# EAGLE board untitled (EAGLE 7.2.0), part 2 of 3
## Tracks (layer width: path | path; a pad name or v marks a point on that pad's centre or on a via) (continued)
N$28  (via drill 0.6) (continued)
  Top 0.406: R20.1 38.1,123.19 38.1,120.65 35.56,119.38 35.56,110.49 R18.1 | C7.2 66.04,110.49 63.5,107.95 v52.07,107.95 U1.18 52.07,101.6 54.61,99.06 U1.4 54.61,93.98 53.34,92.71 U$1.3 | R46.1 100.33,121.92 102.87,120.65 102.87,119.38 101.6,118.11 101.6,110.49 R44.1 | U2.4 109.22,99.06 109.22,104.46 U2.18 v107.95,109.22 | R67.1 146.05,123.19 146.05,110.49 R65.1 | v152.4,109.22 U3.18 152.4,102.87 154.94,100.33 U3.4 | R89.1 201.93,111.76 R87.1 208.28,109.22 v210.82,106.68 | v229.87,106.68 U4.18 229.87,102.87 232.41,100.33 U4.4
  Bottom 0.406: R18.1 38.1,107.95 v52.07,107.95 | U$1.3 56.83,88.9 R22.1 63.5,93.98 R24.2 | C7.2 93.98,111.76 96.52,109.22 R44.1 v107.95,109.22 109.22,110.49 146.05,110.49 R65.1 v152.4,109.22 153.67,110.49 203.2,110.49 R87.1 | v210.82,106.68 v229.87,106.68
N$29  (via drill 0.6)
  Top 0.406: v52.07,125.73 IC3.8 52.07,119.38 50.8,118.11 50.8,106.68 U1.19
  Bottom 0.406: R19.1 38.1,125.73 v52.07,125.73
N$30
  Top 0.406: R19.2 R20.2
  Bottom 0.406: R21.1 R20.2 41.91,124.46 IC3.13
N$31  (via drill 0.6)
  Top 0.406: IC2.6 v62.23,127 v57.15,127 57.15,124.46 R21.2
  Bottom 0.406: IC3.14 38.1,120.65 62.23,120.65 62.23,123.19 60.96,124.46 R21.2
N$32  (via drill 0.6)
  Top 0.406: IC3.2 39.37,113.03 43.18,109.22 43.18,102.87 44.45,101.6 v44.45,96.52
  Bottom 0.406: v44.45,96.52 48.26,96.52 U1.2
N$33
  Top 0.406: IC3.9 49.53,119.38 48.26,118.11 48.26,107.95 46.99,106.68 U1.20
N$34
  Top 0.406: C9.1 R25.2
  Bottom 0.61: IC3.4 45.72,115.57 57.15,115.57 C9.1
N$35
  Bottom 0.406: U$1.1 55.56,87.63 59.69,87.63 60.96,88.9 R22.2 R23.1
N$36
  Bottom 1.422: D12.C D10.A 123.19,149.86 IC4.15 118.11,149.86 118.11,162.56 121.92,167.64 X2.2
N$37
  Bottom 0.406: 138.43,149.86 IC5.1
  Bottom 1.422: IC5.1 133.35,149.86 D13.A D15.C | X2.3 124.46,162.56 127,160.02 137.16,160.02 138.43,158.75 138.43,149.86
N$38
  Top 0.406: C8.1 R26.2
  Bottom 0.406: C8.1 57.15,123.19 45.72,123.19 IC3.11
N$39
  Top 1.422: IC5.15 165.1,149.86 D14.A D16.C
  Bottom 1.422: X2.4 127,167.64 128.27,162.56 152.4,162.56 158.75,154.94 158.75,149.86 IC5.15
N$40
  Top 1.422: IC5.14 R30.1 166.37,154.94 D14.C
N$41
  Top 1.422: R29.1 IC5.2
  Bottom 1.422: D13.C 132.08,154.94 R29.1
N$42
  Top 1.422: D9.A 91.44,149.86 IC4.1
  Bottom 1.422: D11.C D9.A | IC4.1 97.79,151.13 97.79,157.48 99.06,158.75 110.49,158.75 119.38,168.91 X2.1
N$43
  Top 1.422: R28.1 IC4.14
  Bottom 1.422: D10.C 124.46,154.94 R28.1
N$44
  Top 1.422: D9.C 90.17,154.94 R27.1 IC4.2
N$45  (via drill 0.6)
  Top 0.406: IC4.13 R31.2 115.57,143.51 116.84,142.24 116.84,137.16 120.65,133.35 v123.19,133.35 | v153.67,133.35 153.67,137.16 154.94,138.43 IC5.13
  Bottom 0.406: v123.19,133.35 137.16,133.35 139.7,132.08 148.59,132.08 151.13,133.35 v153.67,133.35
N$46
  Top 0.406: R34.1 IC4.11
  Bottom 0.406: R34.1 110.49,142.24 110.49,139.7 R33.2
N$47  (via drill 0.6)
  Top 0.406: IC4.4 v102.87,152.4 | v106.68,152.4 107.95,151.13 107.95,142.24 109.22,140.97 R34.2 113.03,139.7 C11.2
  Bottom 0.406: v102.87,152.4 v106.68,152.4
N$48
  Top 0.406: C11.1 139.7,132.08 | C12.2 139.7,132.08 | 139.7,132.08 139.7,144.78 143.51,148.59 IC5.4
  Bottom 0.406: IC5.10 149.86,156.21 144.78,156.21 IC5.4
N$49
  Top 0.406: R35.2 IC5.11
N$50
  Top 0.406: OK1.1 R93.2
N$51
  Top 0.406: IC4.5 104.14,148.59 101.6,146.05 R36.2
N$52
  Bottom 0.406: R37.1 R36.1 C13.2
N$53
  Top 0.406: R38.2 IC4.7
  Bottom 0.406: R37.2 R38.2
N$54
  Bottom 0.406: C14.1 R38.1
N$55
  Top 0.406: C14.2 IC4.9
N$56
  Top 0.406: R39.2 142.24,146.05 144.78,148.59 IC5.5
N$57
  Top 0.406: C15.2 R39.1
  Bottom 0.406: R40.1 R39.1
N$58
  Top 0.406: IC5.7 R41.2
  Bottom 0.406: R40.2 R41.2
N$59
  Top 0.406: R41.1 C16.1
N$60
  Top 0.406: IC5.9 C16.2
N$61  (via drill 0.6)
  Top 0.406: IC4.6 v105.41,129.54 | R42.2 120.65,111.76 IC6.7 119.38,115.57 v119.38,127 118.11,128.27 115.57,128.27 v114.3,127 v111.76,129.54
  Bottom 0.406: v105.41,129.54 v111.76,129.54
N$62
  Top 0.406: R42.1 IC6.6 | R44.2 R43.2
  Bottom 0.406: R43.2 R42.1
N$63  (via drill 0.6)
  Top 0.406: R43.1 IC6.1 | U2.3 106.68,99.06 v106.68,111.76
  Bottom 0.406: v106.68,111.76 R43.1
N$64
  Bottom 0.406: R95.1 45.72,176.53 45.72,174.3 X1.9
N$65  (via drill 0.6)
  Top 0.406: IC6.8 116.84,123.19 v116.84,127 | U2.19 v105.41,110.49 | R45.1 99.06,125.73 v99.06,110.49
  Bottom 0.406: v116.84,127 116.84,128.27 101.6,128.27 R45.1 | v105.41,110.49 v99.06,110.49
N$66
  Top 0.406: R46.2 R45.2
  Bottom 0.406: IC6.13 105.41,123.19 106.68,124.46 R46.2 111.76,123.19 121.92,123.19 R47.1
N$67  (via drill 0.6)
  Top 0.406: IC5.6 146.05,132.08 143.51,129.54 129.54,129.54 v127,127 v121.92,127
  Bottom 0.406: 113.03,125.73 120.65,125.73 v121.92,127 | R47.2 113.03,125.73 | 113.03,125.73 109.22,125.73 107.95,127 105.41,127 102.87,124.46 IC6.14
N$68
  Top 0.406: IC6.2 104.14,113.03 104.14,99.06 U2.2
N$69  (via drill 0.6)
  Top 0.406: IC6.9 115.57,123.19 v109.22,123.19 | v100.33,120.65 100.33,109.22 102.87,106.68 U2.20
  Bottom 0.406: v109.22,123.19 109.22,120.65 v100.33,120.65
N$70
  Bottom 1.422: D20.C D18.A 207.01,149.86 200.66,149.86 | 200.66,149.86 IC7.15 | X3.2 210.82,166.37 205.74,161.29 204.47,161.29 200.66,157.48 200.66,149.86
N$71
  Bottom 0.406: R51.2 C19.1 124.46,116.84 113.03,116.84 IC6.4
N$72
  Bottom 0.406: R52.2 C18.1 123.19,120.65 111.76,120.65 IC6.11
N$73
  Bottom 1.422: D23.C D21.A 217.17,149.86 222.25,149.86 | IC8.1 222.25,149.86 | 222.25,149.86 222.25,158.75 219.71,161.29 215.9,161.29 213.36,165.1 X3.3
N$74
  Top 1.422: IC8.15 248.92,149.86 D22.A D24.C
  Bottom 1.422: IC8.15 242.57,149.86 242.57,157.48 240.03,160.02 227.33,160.02 223.52,163.83 217.17,163.83 215.9,166.37 X3.4
N$75
  Top 1.422: IC8.14 R50.1 250.19,154.94 D22.C
N$76
  Top 1.422: R49.1 IC8.2
  Bottom 1.422: R49.1 215.9,154.94 D21.C
N$77
  Top 1.422: D19.C D17.A 173.99,149.86 IC7.1
  Bottom 1.422: X3.1 204.47,163.83 201.93,163.83 196.85,158.75 182.88,158.75 180.34,156.21 180.34,149.86 IC7.1
N$78
  Top 1.422: IC7.14 R48.1
  Bottom 1.422: R48.1 208.28,154.94 D18.C
N$79
  Top 1.422: D17.C 173.99,154.94 R32.1 IC7.2
N$80  (via drill 0.6)
  Top 0.406: IC7.13 196.85,146.05 198.12,144.78 R53.2 204.47,143.51 207.01,140.97 v208.28,140.97 | v223.52,152.4 219.71,152.4 217.17,149.86 v217.17,142.24
  Bottom 0.406: IC8.13 236.22,152.4 v223.52,152.4 | v217.17,142.24 215.9,140.97 v208.28,140.97
N$81
  Top 0.406: IC7.11 R54.2 195.58,142.24 195.58,138.43 R55.1
N$82  (via drill 0.6)
  Top 0.406: C17.2 195.58,133.35 R55.2 193.04,135.89 193.04,139.7 190.5,142.24 190.5,151.13 v189.23,152.4
  Bottom 0.406: IC7.4 185.42,153.67 186.69,152.4 v189.23,152.4
N$83
  Top 0.406: IC8.4 224.79,152.4 224.79,134.62 | 224.79,134.62 C21.2 | 224.79,134.62 224.79,133.35 C17.1
  Bottom 0.406: IC8.10 233.68,156.21 228.6,156.21 IC8.4
N$84
  Top 0.406: IC8.11 R56.2
N$85
  Top 0.406: R57.2 184.15,146.05 185.42,147.32 186.69,147.32 IC7.5
N$86
  Bottom 0.406: R58.1 R57.1 C22.2
N$87
  Top 0.406: IC7.7 R59.2
  Bottom 0.406: R58.2 R59.2
N$88
  Top 0.406: C23.1 R59.1
N$89
  Top 0.406: C23.2 IC7.9
N$90
  Top 0.406: R60.2 226.06,144.78 228.6,148.59 IC8.5
N$91
  Top 0.406: R61.1 R60.1
  Bottom 0.406: C24.2 R60.1
N$92
  Top 0.406: R62.2 IC8.7
  Bottom 0.406: R62.2 R61.2
N$93
  Bottom 0.406: C25.1 R62.1
N$94
  Top 0.406: IC8.9 C25.2
N$95  (via drill 0.6)
  Top 0.406: IC7.6 187.96,138.43 182.88,133.35 175.26,133.35 172.72,130.81 161.29,130.81 160.02,129.54 v160.02,127 v165.1,127 163.83,125.73 163.83,115.57 IC9.7
  Bottom 0.406: R63.2 165.1,111.76 IC9.7
N$96
  Top 0.406: R65.2 R64.2
  Bottom 0.406: IC9.6 R63.1 R64.2
N$97
  Top 0.406: IC9.1 R64.1 148.59,110.49 148.59,101.6 U3.3
N$98  (via drill 0.6)
  Top 0.406: R66.1 158.75,125.73 162.56,125.73 IC9.8 | v151.13,123.51 151.13,120.65 149.86,120.65 148.59,119.38 148.59,113.03 149.86,111.76 U3.19
  Bottom 0.406: IC9.8 161.29,123.51 v151.13,123.51
N$99  (via drill 0.5 pad 0.41, 0.6)
  Top 0.406: v149.86,124.46 IC9.13
  Bottom 0.406: R68.1 R67.2 v149.86,124.46 R66.2
N$100  (via drill 0.6)
  Top 0.406: IC8.6 229.87,132.08 228.6,130.81 208.28,130.81 205.74,128.27 199.39,128.27 198.12,127 v171.45,127 | IC9.14 148.59,123.19 148.59,125.73 v151.13,125.73
  Bottom 0.406: R68.2 168.91,125.73 167.64,125.73 | 167.64,125.73 v167.64,127 v171.45,127 | v151.13,125.73 167.64,125.73
N$101
  Top 0.406: U3.2 151.13,96.52 153.03,96.52 153.67,97.47 153.67,99.06 151.13,101.6 151.13,113.03 IC9.2
N$102  (via drill 0.6)
  Top 0.406: U3.20 144.78,107.95 v144.78,123.19
  Bottom 0.406: IC9.9 160.02,122.87 152.4,122.87 151.45,122.56 150.81,122.56 150.18,122.87 149.86,123.19 v144.78,123.19
N$103
  Bottom 0.406: IC9.4 156.21,115.57 167.64,115.57 C27.1 R69.2
N$104
  Bottom 0.406: IC9.11 156.21,120.65 167.64,120.65 C26.1 R70.2
N$105
  Bottom 1.016: D26.A D28.C
  Bottom 1.422: D26.A 290.83,149.86 285.75,149.86 | 285.75,149.86 IC10.15 | 285.75,149.86 285.75,160.02 292.1,166.37 292.1,171.25 X4.2
N$106
  Bottom 1.016: D29.A D31.C
  Bottom 1.422: D29.A 300.99,149.86 306.07,149.86 | IC11.1 306.07,149.86 | 306.07,149.86 306.07,157.48 303.53,160.02 298.45,160.02 294.64,166.37 X4.3
N$107
  Top 1.016: D30.A D32.C
  Top 1.422: IC11.15 331.47,149.86 D30.A
  Bottom 1.422: IC11.15 326.39,149.86 326.39,157.48 325.12,158.75 309.88,158.75 306.07,162.56 299.72,162.56 297.18,166.37 X4.4
N$108
  Top 1.422: IC11.14 R74.1 332.74,154.94 D30.C
N$109
  Top 1.422: R73.1 IC11.2
  Bottom 1.422: R73.1 299.72,154.94 D29.C
N$110
  Top 1.422: IC10.1 265.43,151.13 257.81,151.13 D25.A
  Bottom 1.016: D27.C D25.A
  Bottom 1.422: IC10.1 265.43,149.86 265.43,156.21 267.97,158.75 279.4,158.75 X4.1
N$111
  Top 1.422: D26.C 292.1,154.94 R72.1 IC10.14
N$112
  Top 1.422: D25.C 257.81,154.94 R71.1 IC10.2
N$113  (via drill 0.6)
  Top 0.406: IC10.13 R75.2 283.21,143.51 v283.21,137.16 | IC11.13 v322.58,142.24
  Bottom 0.406: v322.58,142.24 308.61,142.24 307.34,140.97 307.34,138.43 304.8,135.89 288.29,135.89 287.02,137.16 v283.21,137.16
N$114
  Top 0.406: IC10.11 R76.2
  Bottom 0.406: R76.2 280.67,142.24 280.67,139.7 R77.1
N$115  (via drill 0.6)
  Top 0.406: IC10.4 270.51,148.59 267.97,144.78 v267.97,135.89 | C29.2 R77.2
  Bottom 0.406: v267.97,135.89 R77.2
N$116
  Top 0.406: C30.2 311.15,137.16 311.15,144.78 313.69,147.32 313.69,151.13 311.15,153.67 IC11.4
  Bottom 0.406: C29.1 306.07,132.08 C30.2 | IC11.10 317.5,153.67 312.42,153.67 IC11.4
N$117
  Top 0.406: IC11.11 R78.2
N$118
  Top 0.406: IC10.5 271.78,148.59 269.24,144.78 R79.2
N$119
  Bottom 0.406: R80.1 R79.1 C31.2
N$120
  Top 0.406: IC10.7 R81.2
  Bottom 0.406: R80.2 R81.2
N$121
  Bottom 0.406: R81.1 C32.1
N$122
  Top 0.406: IC10.9 C32.2
N$123
  Top 0.406: IC11.5 312.42,147.32 309.88,144.78 R82.2
N$124
  Bottom 0.406: R83.1 R82.1 C33.2
N$125
  Top 0.406: IC11.7 R84.2
  Bottom 0.406: R83.2 R84.2
N$126
  Bottom 0.406: C34.1 R84.1
N$127
  Top 0.406: IC11.9 C34.2
N$128  (via drill 0.6)
  Top 0.406: v219.71,111.76 IC12.7 220.98,115.57 220.98,125.73 v219.71,127 v214.63,127 | v273.05,128.27 IC10.6
  Bottom 0.406: v219.71,111.76 R85.2 | v214.63,127 214.63,128.27 215.9,129.54 271.78,129.54 v273.05,128.27
N$129
  Top 0.406: R86.2 R87.2 | IC12.6 R85.1
  Bottom 0.406: R86.2 R85.1
N$130  (via drill 0.6)
  Top 0.406: IC12.1 R86.1 208.28,111.76 v212.09,107.95 | v228.6,107.95 228.6,99.06 U4.3
  Bottom 0.406: v212.09,107.95 v228.6,107.95
N$131  (via drill 0.6)
  Top 0.406: IC12.8 218.44,120.65 v218.44,104.14
  Bottom 0.406: R88.1 203.2,125.73 203.2,120.65 218.44,120.65 IC12.8 | v218.44,104.14 226.06,104.14 U4.19
N$132
  Top 0.406: R88.2 R89.2 209.55,124.46 IC12.13
  Bottom 0.406: R89.2 R90.1
N$133  (via drill 0.6)
  Top 0.406: IC11.6 313.69,153.67 314.96,152.4 316.23,152.4 316.23,134.62 v306.07,125.73 | IC12.14 204.47,125.73 207.01,128.27 220.98,128.27 v222.25,127 223.52,127 | R90.2 224.79,125.73 223.52,127 | 223.52,127 v227.33,127
  Bottom 0.406: v227.33,127 274.32,127 276.86,125.73 v306.07,125.73
N$134  (via drill 0.6)
  Top 0.406: v227.33,102.87 U4.2
  Bottom 0.406: IC12.2 207.01,106.68 210.82,102.87 v227.33,102.87
N$135  (via drill 0.6)
  Top 0.406: IC12.9 215.9,120.65 v215.9,105.09
  Bottom 0.406: v215.9,105.09 U4.20
N$136
  Top 0.406: C36.1 R91.2
  Bottom 0.406: IC12.4 213.36,113.03 223.52,113.03 C36.1
N$137
  Top 0.406: C35.1 R92.2
  Bottom 0.406: IC12.11 213.36,123.19 223.52,123.19 C35.1
N$138
  Top 0.406: R94.1 24.13,172.72 24.13,176.53 40.64,176.53 40.64,174.09 X1.7
N$139  (via drill 0.6)
  Top 0.406: R97.1 106.05,177.17 115.57,177.17 v116.2,176.53
  Bottom 0.406: v116.2,176.53 127.3,176.53 X2.9
N$140  (via drill 0.6)
  Top 0.406: U2.14 118.11,102.87 119.38,101.6 v119.38,100.01 119.38,85.09 118.11,83.82 v118.11,77.47 | v62.23,100.01 U1.14 | v143.51,77.47 IC13.13 | RN1.2 IC16.2 | v106.68,77.47 v106.68,58.42
  Bottom 0.406: v119.38,100.01 v62.23,100.01 | v143.51,77.47 v118.11,77.47 v106.68,77.47 | IC23.52 v106.68,58.42 106.68,50.8 107.95,49.53 RN1.2
N$141
  Top 0.406: R98.1 233.68,176.53 232.41,177.8 215.8,177.8 X3.7
N$142
  Top 0.406: X3.9 220.98,173.99 222.25,172.72 222.25,168.91 223.52,167.64 233.68,167.64 234.95,168.91 R99.1
N$143  (via drill 0.6)
  Top 0.406: X4.7 293.27,175.36 292.1,176.53 278.13,176.53 275.59,173.99 R100.1 | JP2.1 267.97,177.8 270.51,175.26 v270.51,171.45
  Bottom 0.406: v270.51,171.45 271.78,170.18 274.32,170.18 R100.1
N$144
  Top 0.406: X4.9 298.45,174.3 298.45,175.26 295.91,177.8 276.86,177.8 R101.1
N$145  (via drill 0.6)
  Top 0.406: v243.84,148.59 243.84,144.78 240.03,140.97 v240.03,124.46
  Bottom 0.406: R99.2 243.84,162.56 v243.84,148.59 | v240.03,124.46 252.73,124.46 OK4.1
N$146  (via drill 0.6)
  Top 0.406: R98.2 246.38,176.53 250.19,172.72 250.19,166.37 251.46,165.1 v251.46,163.83 | v252.73,137.16 252.73,124.46 OK4.3
  Bottom 0.406: v251.46,163.83 252.73,161.29 v252.73,137.16
N$147  (via drill 0.6)
  Top 0.406: v11.43,147.32 11.43,144.78 15.24,140.97 v15.24,135.89
  Bottom 0.406: R95.2 21.59,175.26 21.59,162.56 20.32,161.29 13.97,161.29 12.7,160.02 12.7,153.67 11.43,152.4 v11.43,147.32 | v15.24,135.89 19.05,132.08 72.39,132.08 80.01,124.46 OK2.1
N$148
  Bottom 0.406: R94.2 15.24,171.45 13.97,170.18 7.62,170.18 5.08,167.64 5.08,135.89 10.16,130.81 71.12,130.81 74.93,127 OK2.3
N$149
  Bottom 0.406: R97.2 101.6,177.8 92.71,177.8 86.36,171.45 86.36,132.08 92.71,125.73 OK3.1
N$150  (via drill 0.6)
  Top 0.406: R96.2 88.9,171.45 v86.36,173.99
  Bottom 0.406: v86.36,173.99 85.09,172.72 85.09,130.81 86.36,129.54 86.36,127 87.63,125.73 OK3.3
N$151  (via drill 0.6)
  Top 0.406: R101.2 274.32,176.53 274.32,168.91 273.05,167.64 270.51,167.64 269.24,166.37 269.24,163.83 v265.43,163.83 | v264.16,148.59 265.43,147.32 265.43,125.73 OK5.1
  Bottom 0.406: v265.43,163.83 264.16,162.56 v264.16,148.59
N$152  (via drill 0.6)
  Top 0.406: R100.2 273.05,170.18 271.78,168.91 269.24,168.91 267.97,167.64 267.97,166.37 264.16,166.37 262.89,165.1 v262.89,163.83 | v262.89,148.59 262.89,147.32 264.16,146.05 OK5.3
  Bottom 0.406: v262.89,163.83 v262.89,148.59
N$153
  Bottom 1.676: F3.2A 16.51,124.46 11.43,119.38 7.62,119.38 5.08,116.84 B1.AC2
N$154
  Bottom 1.676: B1.AC1 10.16,109.22 12.7,106.68 12.7,99.06 X15.2
N$155  (via drill 0.6)
  Top 0.406: U2.13 120.65,102.87 121.92,101.6 v121.92,100.01 121.92,85.09 120.65,83.82 v120.65,78.74 | v64.77,100.97 U1.13 | IC13.14 v146.05,78.74 | RN1.3 IC16.3 | v105.41,78.74 v105.41,57.15 106.68,55.88 v106.68,46.99
  Bottom 0.406: v121.92,100.01 120.02,100.97 119.06,100.97 118.43,100.65 65.41,100.65 v64.77,100.97 | v146.05,78.74 v120.65,78.74 v105.41,78.74 | IC23.51 95.25,57.15 v105.41,57.15 | v106.68,46.99 RN1.3
N$156  (via drill 0.6)
  Top 0.406: U2.12 123.19,102.87 124.46,101.6 v124.46,100.01 124.46,85.09 123.19,83.82 v123.19,80.01 | v67.31,101.6 U1.12 | v148.59,80.01 IC13.15 | RN1.4 IC16.4 | v104.14,80.01 v104.14,55.88 105.41,54.61 105.41,45.72 v106.68,44.45
  Bottom 0.406: v124.46,100.01 121.92,101.6 118.75,101.6 118.11,101.28 67.95,101.28 v67.31,101.6 | v148.59,80.01 v123.19,80.01 v104.14,80.01 | IC23.50 v104.14,55.88 | v106.68,44.45 RN1.4
N$157  (via drill 0.6)
  Top 0.406: v127,95.57 v127,102.24 125.73,102.87 U2.11 | v151.13,95.57 IC13.17 | v69.85,102.24 U1.11 | IC16.5 RN1.5 107.31,41.91 104.78,44.45 104.78,52.71 v102.87,54.61 v102.87,95.57
  Bottom 0.406: v127,102.24 118.43,102.24 117.79,101.92 70.17,101.92 v69.85,102.24 | v151.13,95.57 146.68,95.57 146.05,96.2 130.49,96.2 129.86,95.57 v127,95.57 v102.87,95.57 | IC23.49 95.25,54.61 v102.87,54.61
N$158  (via drill 0.6)
  Top 0.406: U2.10 v125.73,94.62 | IC13.18 148.59,90.17 149.86,91.44 v149.86,94.62 | IC16.6 RN1.6 107.31,39.37 104.14,42.55 104.14,50.8 v102.23,53.34 101.6,53.98 v101.6,94.62
  Bottom 0.406: v149.86,94.62 149.54,94.93 130.81,94.93 130.49,94.62 v125.73,94.62 v101.6,94.62 84.14,94.62 81.28,97.79 U1.10 | IC23.48 v102.23,53.34
N$159  (via drill 0.6)
  Top 0.406: U2.9 v123.19,93.66 | v100.33,93.66 100.33,93.34 100.97,92.71 v100.97,52.07 103.5,49.53 103.5,40.64 107.31,36.83 RN1.7 IC16.7 | IC13.19 144.78,90.17 143.51,90.17 142.24,91.44 140.97,91.44 139.7,92.71 v139.7,93.66
  Bottom 0.406: U1.9 68.58,96.52 80.01,96.52 82.55,93.66 v100.33,93.66 v123.19,93.66 v139.7,93.66 | IC23.47 95.25,52.07 v100.97,52.07
N$160  (via drill 0.6)
  Top 0.406: U2.8 v120.65,91.44 | v62.23,95.25 U1.8 | IC16.8 RN1.8 107.31,34.29 102.87,38.74 102.87,47.63 v100.01,50.8 v100.01,91.44
  Bottom 0.406: IC13.20 140.97,91.44 v120.65,91.44 v100.01,91.44 81.92,91.44 78.42,95.25 v62.23,95.25 | IC23.46 v100.01,50.8
N$161  (via drill 0.6)
  Top 0.406: U2.7 v118.11,92.71 | IC13.21 v137.16,92.71 | RN1.9 IC16.9 | v99.06,92.71 v99.06,49.53 99.06,33.66 99.7,33.02 v100.33,33.02
  Bottom 0.406: v137.16,92.71 v118.11,92.71 v99.06,92.71 81.92,92.71 79.06,95.89 64.14,95.89 U1.7 | IC23.45 95.25,49.53 v99.06,49.53 | v100.33,33.02 101.6,31.75 RN1.9
N$162  (via drill 0.6)
  Top 0.406: IC17.18 186.69,101.6 v187.64,100.97 | U3.14 161.29,103.82 v161.29,102.87 161.29,90.17 160.66,88.58 160.66,61.6 v161.29,60.96 160.66,60.33 v160.66,39.37 | IC19.11 200.34,57.15 v200.34,58.42 | U4.14 240.03,102.87 238.76,101.6 238.76,91.44 237.49,90.17 v237.49,77.47 | IC21.3 226.06,76.2 224.47,74.61 v224.47,57.15 | v187.96,55.88 187.96,43.18 IC18.18
  Bottom 0.406: v187.64,100.97 186.69,101.6 162.56,101.6 v161.29,102.87 | v200.34,58.42 199.39,58.42 198.12,57.15 190.5,57.15 189.23,55.88 v187.96,55.88 IC14.13 | v237.49,77.47 233.68,77.47 232.41,76.2 IC21.3 | v224.47,57.15 223.52,57.15 220.98,54.61 209.55,54.61 208.28,55.88 IC19.11 | IC18.18 184.15,39.37 v160.66,39.37 | v161.29,60.96 156.21,60.96 154.94,62.23 IC20.2 RN4.2 114.3,62.23 107.95,68.58 IC23.60
N$163  (via drill 0.6)
  Top 0.406: IC18.17 v189.23,53.34 | v211.77,52.07 211.77,41.91 v209.55,39.37 | IC21.4 227.01,73.66 225.42,72.07 225.42,57.79 226.06,57.15 226.06,54.93 v225.74,54.61 | v239.39,74.93 240.03,75.57 240.03,90.17 241.3,91.44 241.3,101.6 242.57,102.87 U4.13 | v178.12,53.34 v178.12,58.42 | U3.13 165.1,101.6 163.83,100.33 163.83,93.03 164.46,92.39 164.46,64.14 163.51,63.18 163.51,58.74 v163.19,58.42
  Bottom 0.406: v189.23,53.34 IC14.14 v178.12,53.34 | IC19.12 208.28,53.34 209.55,52.07 v211.77,52.07 220.98,52.07 223.52,54.61 v225.74,54.61 | v209.55,39.37 204.47,39.37 203.2,40.64 190.5,40.64 IC18.17 | IC17.17 187.96,106.36 166.05,106.36 U3.13 | IC21.4 232.41,73.66 233.68,74.93 v239.39,74.93 | v178.12,58.42 v163.19,58.42 156.21,58.42 154.94,59.69 IC20.3 RN4.3 113.67,59.69 113.03,60.33 113.03,62.23 107.95,67.31 95.25,67.31 IC23.59
N$164  (via drill 0.6)
  Top 0.406: v190.5,50.8 v190.5,48.26 190.5,44.45 191.77,43.18 IC18.16 | IC21.7 226.38,63.82 226.38,58.1 227.01,57.47 227.01,53.34 v228.28,52.07 | U4.12 245.11,102.87 243.84,101.6 243.84,91.44 241.3,88.9 v241.3,67.31 | 174.62,104.14 v174.62,105.41 174.62,85.09 173.67,84.14 173.67,56.83 v172.72,55.88 v172.72,52.07
  Bottom 0.406: U3.12 168.91,104.14 175.26,104.14 | IC17.16 190.5,104.14 175.26,104.14 | v190.5,48.26 193.04,48.26 194.31,49.53 198.12,49.53 199.39,50.8 IC19.13 208.28,50.8 209.55,49.53 222.25,49.53 224.79,52.07 v228.28,52.07 | v190.5,50.8 IC14.15 173.99,50.8 v172.72,52.07 | v241.3,67.31 233.68,67.31 232.41,66.04 IC21.7 | 175.26,104.14 v174.62,105.41 | v172.72,55.88 156.21,55.88 154.94,57.15 IC20.4 RN4.4 124.46,57.15 123.83,57.79 113.67,57.79 112.39,59.06 112.39,61.6 107.95,66.04 IC23.58
N$165  (via drill 0.6, 0.6 pad 0.61)
  Top 0.406: IC17.15 194.31,102.87 193.04,101.6 193.04,92.71 194.31,91.44 v194.31,90.17 | v203.2,90.17 v203.2,49.53 | IC14.17 196.85,44.45 IC18.15 193.04,43.18 v193.04,52.07 | U3.11 v170.18,107.31 | IC21.8 227.33,62.23 227.33,58.1 227.96,57.47 227.96,55.88 229.87,53.98 v229.87,53.34 | U4.11 247.65,102.55 246.38,101.28 246.38,91.44 243.84,88.9 243.84,64.45 v243.52,64.14
  Bottom 0.406: v170.18,107.31 192.72,107.31 IC17.15 | v194.31,90.17 v203.2,90.17 | IC14.17 198.12,48.26 199.39,49.53 v203.2,49.53 208.28,49.53 209.55,48.26 IC19.15 222.88,48.26 225.11,50.48 228.92,50.48 229.87,51.44 v229.87,53.34 | v243.52,64.14 237.17,64.14 236.22,64.77 233.68,64.77 232.41,63.5 IC21.8 | v193.04,52.07 175.26,52.07 173.99,53.34 156.21,53.34 154.94,54.61 IC20.5 RN4.5 125.73,54.61 123.19,57.15 113.03,57.15 111.76,58.42 111.76,60.96 107.95,64.77 95.25,64.77 IC23.57
N$166  (via drill 0.6)
  Top 0.406: IC17.14 196.85,102.87 195.58,101.6 v195.58,91.44 | v204.47,91.44 v204.47,52.07 v204.47,45.72 | v232.41,54.93 235.27,54.93 237.49,57.15 237.49,62.23 IC21.13 | U4.10 247.65,90.17 245.11,87.63 v245.11,63.5 | U3.10 170.18,92.71 167.64,90.17 167.64,85.73 168.91,84.46 168.91,80.65 167.32,78.74 v167.32,50.8
  Bottom 0.406: v195.58,91.44 v204.47,91.44 | IC18.14 200.66,45.72 v204.47,45.72 | v232.41,54.93 229.23,54.93 227.01,53.34 223.84,53.34 221.3,50.8 IC19.16 209.55,50.8 208.28,52.07 v204.47,52.07 199.39,52.07 198.12,50.8 IC14.18 194.31,50.8 193.04,49.53 173.04,49.53 171.77,50.8 v167.32,50.8 156.21,50.8 154.94,52.07 IC20.6 RN4.6 125.73,52.07 124.46,53.34 124.46,54.61 122.56,56.52 112.39,56.52 111.12,57.79 111.12,60.33 107.95,63.5 IC23.56 | v245.11,63.5 244.47,62.87 236.85,62.87 IC21.13
N$167  (via drill 0.6)
  Top 0.406: IC17.13 199.39,102.87 200.66,101.6 203.2,101.6 205.74,99.06 v205.74,54.61 v205.74,44.45 | IC21.14 234.95,64.77 234.95,57.47 234.31,56.83 v231.77,56.83 | U4.9 245.11,91.44 242.57,88.9 242.57,66.68 v242.25,66.04 | v191.77,46.99 v191.77,53.02 | U3.9 167.64,94.62 166.37,93.34 166.37,63.5 164.78,61.91 164.78,49.85 165.1,49.53 v165.1,48.26
  Bottom 0.406: IC18.13 201.93,44.45 v205.74,44.45 | v231.77,56.83 228.92,56.83 227.01,55.56 223.2,55.56 220.98,53.34 IC19.17 209.55,53.34 208.28,54.61 v205.74,54.61 199.39,54.61 198.12,53.34 IC14.19 193.99,53.34 192.72,53.02 v191.77,53.02 | v242.25,66.04 240.66,66.04 240.03,66.68 237.17,66.68 IC21.14 | v191.77,46.99 179.07,46.99 177.8,48.26 v165.1,48.26 156.21,48.26 154.94,49.53 IC20.7 RN4.7 130.17,49.53 128.91,50.8 125.73,50.8 123.83,52.71 123.83,53.98 121.92,55.88 111.76,55.88 110.49,57.15 110.49,59.69 107.95,62.23 95.25,62.23 IC23.55
N$168  (via drill 0.6)
  Top 0.406: IC17.12 201.93,104.14 203.2,102.87 204.47,102.87 207.01,100.33 v207.01,57.15 v207.01,41.91 | v223.2,58.1 v223.2,72.39 | U4.8 242.57,91.44 240.66,89.54 240.66,73.98 v240.35,73.66 | v195.58,45.72 195.58,54.61 IC14.20 | v164.15,45.72 164.15,62.55 165.42,63.82 165.42,97.47 U3.8
  Bottom 0.406: IC14.20 198.12,55.88 199.39,57.15 v207.01,57.15 208.28,57.15 209.55,55.88 IC19.18 220.66,55.88 222.88,58.1 v223.2,58.1 | IC18.12 203.2,43.18 205.74,43.18 v207.01,41.91 | v223.2,72.39 232.41,72.39 233.68,73.66 IC21.17 v240.35,73.66 | v195.58,45.72 v164.15,45.72 156.21,45.72 154.94,46.99 IC20.8 RN4.8 128.27,46.99 123.19,52.07 123.19,53.34 121.28,55.25 111.12,55.25 109.86,56.52 109.86,59.06 107.95,60.96 IC23.54
N$169  (via drill 0.6)
  Top 0.406: v209.55,59.69 v209.55,41.91 | U4.7 240.03,91.44 238.76,90.17 238.76,76.84 v238.12,76.2 | v221.93,74.93 v221.93,60.96 | v163.83,102.87 162.56,101.6 U3.7 | v152.4,94.3 152.4,80.01 149.86,77.47 149.86,71.12 148.59,69.85 148.59,46.99 RN4.9 | v194.31,43.5 194.31,55.88 IC14.21 | v107.95,59.06 v107.95,43.18
  Bottom 0.406: IC17.11 204.47,102.87 v163.83,102.87 | v209.55,41.91 208.6,40.64 205.42,40.64 IC18.11 | IC14.21 198.12,58.42 199.39,59.69 v209.55,59.69 210.82,58.42 IC19.19 219.39,58.42 v221.93,60.96 | v238.12,76.2 IC21.18 233.68,76.2 232.41,74.93 v221.93,74.93 | U3.7 162.56,96.52 160.34,94.3 v152.4,94.3 | v194.31,43.5 193.67,43.18 156.21,43.18 154.94,44.45 IC20.9 RN4.9 133.35,44.45 132.08,43.18 v107.95,43.18 | IC23.53 95.25,59.69 107.31,59.69 v107.95,59.06
N$170  (via drill 0.6)
  Top 0.406: IC21.11 236.22,57.15 234.95,55.88 231.77,55.88 230.82,54.93 230.82,52.39 228.92,50.48 224.47,50.48 219.71,45.72 v219.71,26.67
  Bottom 0.406: v219.71,26.67 219.71,24.13 217.8,22.23 170.81,22.23 168.59,20 162.56,20 162.56,17.78 160.02,17.78 IC15.5
N$171  (via drill 0.6)
  Top 0.406: U4.6 237.49,91.44 236.22,90.17 v236.22,89.85 | v219.71,88.9 219.71,83.82 220.98,82.55 220.98,80.01 220.34,78.74 v220.34,62.23 | U3.6 v160.02,91.44 | v140.97,60.96 IC13.12 140.97,82.55 142.24,83.82 142.24,90.17 140.97,90.17 v138.43,92.71 v138.43,97.79
  Bottom 0.406: v236.22,89.85 220.66,89.85 v219.71,88.9 | v220.34,62.23 212.09,62.23 210.82,60.96 IC19.9 199.39,60.96 198.12,59.69 187.96,59.69 186.69,58.42 IC14.12 179.7,58.42 178.75,59.37 162.88,59.37 162.56,59.69 IC20.18 156.21,59.69 154.94,60.96 v140.97,60.96 | v138.43,97.79 115.57,97.79 | U1.6 60.96,99.06 63.5,99.06 63.82,99.38 113.98,99.38 115.57,97.79 | 115.57,97.79 U2.6 | v138.43,92.71 138.75,92.39 141.29,92.39 143.51,90.17 158.75,90.17 v160.02,91.44
N$172
  Top 0.406: U3.15 160.02,101.6 158.75,100.33 158.75,85.09 160.02,83.82 160.02,41.59 159.7,41.28 159.7,39.37 158.75,38.42 158.75,34.29 157.48,34.29 157.48,22.86 IC15.10
  Bottom 0.406: U1.15 60.64,106.36 159.07,106.36 U3.15
N$173  (via drill 0.6)
  Top 0.406: U2.15 115.57,102.87 116.84,101.6 116.84,86.36 115.57,85.09 115.57,76.2 114.3,74.93 v114.3,60.96 | U4.15 233.68,101.28 233.68,95.25 v229.87,91.44 | v212.09,91.44 212.09,53.34 213.36,52.07 213.36,42.23 v209.55,37.78 | IC15.9 v156.21,31.75 | v137.48,31.75 v137.48,60.96
  Bottom 0.406: v229.87,91.44 v212.09,91.44 | v209.55,37.78 209.55,35.56 207.01,33.02 187.01,33.02 185.74,32.39 174.94,32.39 173.99,33.02 165.1,33.02 163.83,31.75 v156.21,31.75 v137.48,31.75 | v137.48,60.96 v114.3,60.96
N$174  (via drill 0.6)
  Top 0.406: U2.16 113.03,102.87 114.3,101.6 114.3,92.71 115.57,91.44 IC13.31 115.57,87.63 114.3,86.36 114.3,77.15 v113.35,76.2 | IC23.41 91.44,46.67 90.17,47.94 v90.17,76.2
  Bottom 0.406: U1.16 58.42,104.14 69.85,104.14 71.12,102.55 112.39,102.55 113.03,103.19 U2.16 | v113.35,76.2 v90.17,76.2
N$175  (via drill 0.6)
  Top 0.406: U4.16 234.95,106.68 238.76,106.68 238.76,104.14 236.22,101.6 236.22,92.71 234.95,91.44 v234.95,88.9 | v228.6,88.9 228.6,86.36 226.06,83.82 v226.06,78.74 | v218.44,78.74 v218.44,86.36 | U3.16 157.48,104.14 156.21,102.87 v156.21,88.9 v156.21,85.09 | v97.79,90.17 98.42,89.54 98.42,72.39 95.25,69.22 95.25,68.26 94.3,67.31 93.34,67.31 92.08,66.04 v92.08,50.8 | v128.27,10.16 128.27,13.97 127.95,14.29 127.95,21.27 127.64,21.59 v127.64,27.31 | v99.7,27.62 99.7,28.26 97.16,30.8 97.16,39.69 92.39,44.45 90.17,44.45 90.17,46.99 IC23.40 v88.9,50.8
  Bottom 0.406: v234.95,88.9 v228.6,88.9 | v226.06,78.74 v218.44,78.74 IC19.27 | v218.44,86.36 217.17,83.82 IC14.31 184.15,83.82 182.88,85.09 171.45,85.09 168.91,82.55 158.75,82.55 v156.21,85.09 | v156.21,88.9 153.67,88.9 152.4,87.63 137.16,87.63 137.16,90.17 v97.79,90.17 | IC15.28 142.24,8.89 141.29,9.84 133.35,9.84 133.03,9.53 131.76,9.53 131.13,10.16 v128.27,10.16 | v127.64,27.31 100.01,27.31 v99.7,27.62 | v92.08,50.8 v88.9,50.8
N$176  (via drill 0.6)
  Top 0.406: IC13.4 120.65,54.61 119.38,53.34 119.38,38.1 IC16.14 | v136.52,36.83 v136.52,23.5
  Bottom 0.406: IC14.4 177.8,78.74 173.67,74.61 163.51,74.61 163.19,74.93 121.92,74.93 IC13.4 | IC16.14 v136.52,36.83 | v136.52,23.5 136.52,23.18 140.65,19.05 IC15.20
N$177  (via drill 0.6)
  Top 0.406: IC13.5 v123.19,69.85 v123.19,49.53 123.19,40.64 125.41,38.42 v125.41,24.45 | v132.4,24.45 v132.4,10.48
  Bottom 0.406: IC19.25 212.09,73.66 208.28,77.47 187.96,77.47 186.69,76.2 IC14.5 177.8,76.2 174.62,73.03 171.77,73.03 170.5,71.76 169.23,71.76 167.64,70.17 123.51,70.17 v123.19,69.85 | v125.41,24.45 v132.4,24.45 | IC15.27 144.78,10.16 142.24,10.16 141.6,10.8 133.03,10.8 v132.4,10.48 | IC16.19 v123.19,49.53
N$178  (via drill 0.6)
  Top 0.406: v171.45,83.82 170.18,82.55 v170.18,76.2
  Bottom 0.406: IC14.2 R102.1 v171.45,83.82 | v170.18,76.2 116.84,76.2 115.57,74.93 IC13.2 115.57,72.39 114.3,71.12 95.89,71.12 94.61,69.85 93.66,69.85 92.71,68.9 92.71,67.95 90.49,65.72 83.5,65.72 81.28,63.5 IC23.34
N$179  (via drill 0.6)
  Top 0.406: v171.45,81.28 v171.45,76.2
  Bottom 0.406: IC14.3 R103.1 v171.45,81.28 | v171.45,76.2 171.45,75.88 170.81,75.25 163.83,75.25 163.51,75.57 118.75,75.57 118.11,74.93 IC13.3 116.52,72.07 116.52,67.63 SV3.2
N$180  (via drill 0.6)
  Top 0.406: IC13.29 120.65,85.09 119.38,83.82 v119.38,71.12 119.38,54.61 118.11,53.34 118.11,34.29 IC16.12 | v133.67,31.75 v133.67,24.45
  Bottom 0.406: IC14.29 187.96,78.74 186.69,77.47 177.8,77.47 173.99,73.66 171.45,73.66 170.18,72.39 168.91,72.39 167.64,71.12 v119.38,71.12 | IC16.12 v133.67,31.75 | v133.67,24.45 140.97,24.45 IC15.18
N$181  (via drill 0.6)
  Top 0.406: IC13.28 123.19,85.09 121.92,83.82 v121.92,68.9 121.92,35.56 IC16.13 | v143.51,24.13 138.43,29.21 v138.43,34.29
  Bottom 0.406: IC14.28 187.96,76.2 186.69,74.93 177.8,74.93 175.26,72.39 172.08,72.39 170.81,71.12 169.54,71.12 167.96,69.53 124.14,69.53 123.19,68.9 v121.92,68.9 | IC15.19 v143.51,24.13 | v138.43,34.29 IC16.13
N$182  (via drill 0.6)
  Top 0.406: 125.73,63.5 IC13.6 v125.73,45.72 | IC14.6 182.88,72.39 182.88,49.53 180.34,49.53 v180.34,44.45
  Bottom 0.406: IC14.6 186.69,73.66 187.96,74.93 199.39,74.93 200.66,76.2 IC19.3 | v180.34,44.45 IC20.12 156.21,44.45 154.94,45.72 v125.73,45.72
N$183  (via drill 0.6)
  Top 0.406: IC13.25 130.81,85.09 129.54,83.82 v129.54,66.68 v129.54,39.37 v129.54,23.5
  Bottom 0.406: IC14.25 187.96,68.58 186.69,67.31 130.17,67.31 v129.54,66.68 | v129.54,23.5 130.81,23.5 131.44,23.18 135.57,23.18 140.97,17.78 144.78,17.78 IC15.21 | IC16.15 v129.54,39.37
N$184  (via drill 0.6)
  Top 0.406: IC13.23 135.89,85.09 134.62,83.82 v134.62,41.91 v134.62,22.23 | v162.56,64.77 v162.56,87
  Bottom 0.406: IC14.23 187.96,63.5 186.69,62.23 165.1,62.23 v162.56,64.77 | v162.56,87 154.3,87 153.67,86.36 135.89,86.36 IC13.23 | v134.62,22.23 135.57,22.23 141.29,16.51 IC15.22 | IC16.16 v134.62,41.91
N$185  (via drill 0.6)
  Top 0.406: v208.28,72.39 v208.28,63.5 | IC13.26 128.27,85.09 127,83.82 v127,67.31 127,46.04 v128.59,44.45 128.59,21.91 128.91,21.59 v128.91,15.24
  Bottom 0.406: IC19.21 v208.28,63.5 | v208.28,72.39 200.66,72.39 199.39,71.12 IC14.26 187.96,71.12 186.69,69.85 170.18,69.85 168.59,68.26 127.95,68.26 v127,67.31 | IC15.25 144.78,15.24 v128.91,15.24 | IC16.17 v128.59,44.45
N$186  (via drill 0.6)
  Top 0.406: IC13.27 125.73,85.09 124.46,83.82 v124.46,68.26 v124.46,46.99 124.46,44.45 126.36,42.55 126.36,20.64 126.68,20.32 126.68,13.97 127,13.65 v127,10.8
  Bottom 0.406: IC19.24 212.09,71.12 208.28,74.93 200.66,74.93 199.39,73.66 IC14.27 187.96,73.66 186.69,72.39 176.53,72.39 175.89,71.76 172.4,71.76 171.13,70.49 169.86,70.49 168.27,68.9 125.1,68.9 v124.46,68.26 | IC15.26 143.19,11.75 127.95,11.75 v127,10.8 | IC16.18 v124.46,46.99
N$187  (via drill 0.6)
  Top 0.406: 128.27,63.5 IC13.7 v128.27,48.9 | 177.8,69.85 v177.8,71.12 177.8,60.96 177.16,60.33 v177.16,46.99
  Bottom 0.406: IC19.4 200.66,73.66 199.39,72.39 187.96,72.39 186.69,71.12 IC14.7 v177.8,71.12 | v177.16,46.99 IC20.13 156.21,46.99 154.94,48.26 128.91,48.26 v128.27,48.9
N$188  (via drill 0.6)
  Top 0.406: IC13.8 v130.81,50.8 | v171.45,68.58 v171.45,49.53
  Bottom 0.406: IC19.5 200.66,71.12 199.39,69.85 187.96,69.85 186.69,68.58 IC14.8 v171.45,68.58 | v171.45,49.53 IC20.14 156.21,49.53 154.94,50.8 v130.81,50.8
N$189  (via drill 0.6)
  Top 0.406: IC13.9 v133.35,53.34 | v170.18,66.04 v170.18,52.07
  Bottom 0.406: IC19.6 200.66,68.58 199.39,67.31 187.96,67.31 186.69,66.04 IC14.9 v170.18,66.04 | v170.18,52.07 IC20.15 156.21,52.07 154.94,53.34 v133.35,53.34
N$190  (via drill 0.6)
  Top 0.406: IC13.10 v135.89,55.88 | v168.91,63.5 v168.91,54.61
  Bottom 0.406: IC19.7 200.66,66.04 199.39,64.77 187.96,64.77 186.69,63.5 IC14.10 v168.91,63.5 | v168.91,54.61 IC20.16 156.21,54.61 154.94,55.88 v135.89,55.88
N$191  (via drill 0.6)
  Top 0.406: IC13.11 v138.43,58.42 | v166.05,60.96 v166.05,57.15
  Bottom 0.406: IC19.8 200.66,63.5 199.39,62.23 187.96,62.23 186.69,60.96 IC14.11 v166.05,60.96 | v166.05,57.15 IC20.17 156.21,57.15 154.94,58.42 v138.43,58.42
N$192  (via drill 0.6)
  Top 0.406: IC13.24 133.35,85.09 132.08,83.82 v132.08,66.04 | v142.24,66.04 v142.24,41.91 | IC18.19 186.69,44.45 186.69,66.04 187.96,67.31 | IC17.19 184.15,100.33 185.42,99.06 185.42,91.44 187.96,88.9 187.96,67.31 | IC14.24 195.58,67.31 187.96,67.31
  Bottom 0.406: IC14.24 199.39,66.04 200.66,67.31 209.55,67.31 210.82,66.04 IC19.22 | v132.08,66.04 v142.24,66.04 | v142.24,41.91 148.59,41.91 149.86,40.64 182.88,40.64 IC18.19
N$193  (via drill 0.6)
  other vias: 93.98,165.1
N$194
  pour Top: 173.99,163.19 175.89,163.19 175.89,164.78 173.99,164.78
N$195  (via drill 0.6)
  other vias: 190.5,163.83
N$196
  Bottom 1.676: X15.6 11.43,80.01 39.37,80.01 40.64,81.28 44.45,81.28 B2.AC1
N$197  (via drill 0.6)
  Top 0.406: IC17.9 RN2.9 | OK5.8 267.97,113.03 265.43,113.03 264.16,111.76 261.62,111.76 260.35,107.95 260.35,97.79 v256.54,93.98
  Bottom 0.406: v256.54,93.98 RN2.9
N$198  (via drill 0.6)
  Top 0.406: IC17.8 RN2.8 | OK5.6 262.89,113.03 260.35,113.03 257.81,109.22 257.81,97.79 v252.73,92.71
  Bottom 0.406: v252.73,92.71 200.66,92.71 RN2.8
N$199  (via drill 0.6)
  Top 0.406: IC17.7 RN2.7 | OK4.8 254,113.03 254,97.79 v252.09,95.89
  Bottom 0.406: v252.09,95.89 198.44,95.89 RN2.7
N$200  (via drill 0.6)
  Top 0.406: IC17.6 RN2.6 | OK4.6 250.19,111.76 251.46,110.49 v251.46,97.79
  Bottom 0.406: v251.46,97.79 250.19,96.52 195.58,96.52 IC17.6
N$201  (via drill 0.6)
  Top 0.406: RN2.5 IC17.5 191.77,101.6 190.5,102.87 v190.5,112.4 | OK3.8 v92.71,109.22 | v143.51,109.22 v143.51,115.57
  Bottom 0.254: v92.71,109.22 93.34,108.27 143.51,108.27 v143.51,109.22 | v143.51,115.57 143.51,116.21 172.72,116.21 172.72,113.67 173.99,112.4 v190.5,112.4
N$202  (via drill 0.6)
  Top 0.406: OK3.6 v87.63,109.22 | v187.96,109.54 187.96,102.87 189.23,101.6 IC17.4 RN2.4 v189.23,90.17 | v181.61,90.17 179.07,87.63 179.07,52.07 178.43,51.44 178.43,46.36 177.8,45.72 v177.8,41.91 | v167.64,41.91 167,41.28 167,29.85 166.37,29.21 v166.37,8.89
  Bottom 0.254: v87.63,109.22 88.9,107.95 168.27,107.95 169.86,109.54 v187.96,109.54
  Bottom 0.406: v189.23,90.17 v181.61,90.17 | v177.8,41.91 v167.64,41.91 | v166.37,8.89 165.1,8.89 162.56,6.35 IC15.39
N$203  (via drill 0.6)
  Top 0.406: RN2.3 IC17.3 186.69,99.06 185.42,100.33 v185.42,108.9 | OK2.8 86.36,110.49 v86.36,109.22
  Bottom 0.254: v86.36,109.22 87.63,107.63 168.59,107.63 169.86,108.9 v185.42,108.9
N$204  (via drill 0.6)
  Top 0.406: RN2.2 IC17.2 184.15,99.06 182.88,100.33 v182.88,108.27 | OK2.6 76.84,112.4 81.92,112.4 85.09,110.49 v85.09,109.22
  Bottom 0.254: v85.09,109.22 86.36,107.31 168.91,107.31 169.86,108.27 v182.88,108.27
N$205  (via drill 0.6)
  Top 0.406: IC19.10 200.66,59.69 199.39,59.69 199.39,60.96 198.12,62.23 191.77,62.23 190.5,63.5 v190.5,66.04
  Bottom 0.406: v190.5,66.04 187.96,66.04 186.69,64.77 168.91,64.77 167.64,66.04 161.29,66.04 160.02,64.77 160.02,63.5 IC20.19
N$206  (via drill 0.6)
  Top 0.406: IC20.11 157.48,40.64 157.48,35.88 156.21,34.61 v154.94,34.61 | v148.59,34.61 v148.59,29.21 | v116.84,29.21 116.52,29.53 116.52,54.93 107.95,63.5 v107.95,81.28 | v93.98,80.65 93.98,75.57 95.25,74.3 95.25,70.49 93.98,69.22 IC23.62
  Bottom 0.406: v154.94,34.61 v148.59,34.61 | v148.59,29.21 IC16.11 v116.84,29.21 | v107.95,81.28 97.79,81.28 C72.2 v93.98,80.65
N$207  (via drill 0.6)
  Top 0.406: IC19.23 215.9,67.31 v215.9,27.31 | v168.91,22.86 v168.91,12.7
  Bottom 0.406: v215.9,27.31 214.63,26.67 214.63,23.5 169.54,23.5 v168.91,22.86 | v168.91,12.7 160.02,12.7 IC15.43
N$208  (via drill 0.6)
  Top 0.406: IC19.20 218.44,59.69 218.44,46.99 217.17,45.72 217.17,27.94 v218.44,26.67
  Bottom 0.406: v218.44,26.67 218.44,24.77 216.53,22.86 170.5,22.86 168.27,20.64 162.24,20.64 161.92,20.32 159.7,20.32 IC15.8
N$209
  Bottom 0.406: OK6.1 172.72,16.51 175.26,13.97 R104.1
N$210  (via drill 0.6)
  Top 0.406: v163.51,80.01 163.51,64.14 162.88,63.5 162.88,59.69 162.24,59.06 v162.24,27.94 | v149.86,27.62 149.86,22.86 IC15.16 | IC23.43 98.42,41.28 98.42,33.02 v100.33,31.12
  Bottom 0.406: IC19.1 199.39,81.28 198.12,82.55 170.18,82.55 170.18,80.01 v163.51,80.01 | v162.24,27.94 161.92,27.94 161.61,27.62 v149.86,27.62 149.86,29.85 148.91,30.8 121.6,30.8 121.28,30.48 100.97,30.48 v100.33,31.12
N$211  (via drill 0.6)
  Top 0.406: v175.26,80.01 175.26,73.34 174.31,72.39 174.31,31.43 v173.99,31.12 | v165.1,31.12 165.1,20.64 164.46,20 v164.46,11.43
  Bottom 0.406: IC19.2 199.39,78.74 198.12,80.01 v175.26,80.01 | v173.99,31.12 173.67,31.43 169.54,31.43 168.59,30.48 165.73,30.48 v165.1,31.12 | IC15.41 160.02,10.16 162.56,10.16 163.83,11.43 v164.46,11.43
N$212  (via drill 0.6)
  Top 0.406: IC13.22 v138.43,85.09 138.43,78.74 139.7,77.47 139.7,31.75 146.05,25.4 IC15.17 | v161.61,86.04 161.61,63.18 v161.92,62.87
  Bottom 0.406: v138.43,85.09 153.67,85.09 154.62,86.04 v161.61,86.04 | v161.92,62.87 165.1,60.01 179.7,60.01 180.02,59.69 186.69,59.69 187.96,60.96 IC14.22
N$213  (via drill 0.6)
  Top 0.406: IC18.9 RN3.9 | v210.82,30.48 213.36,27.94 OK7.6 | IC23.33 83.82,43.18 v83.82,22.86 | v92.71,22.54 v92.71,15.24 | v107.95,15.24 107.95,2.54 109.22,1.27 161.29,1.27 167.64,7.62 v167.64,21.59
  Bottom 0.406: RN3.9 v210.82,30.48 | v83.82,22.86 84.14,22.54 v92.71,22.54 | v92.71,15.24 v107.95,15.24 | v167.64,21.59 167.64,22.86 168.91,24.13 212.09,24.13 OK7.6
N$214  (via drill 0.6)
  Top 0.406: IC18.8 RN3.8 199.39,28.26 v200.34,28.26 | v140.97,38.1 v140.97,33.66 | v163.19,32.7 v163.19,25.72
  Bottom 0.406: OK7.7 210.82,26.67 208.91,28.26 v200.34,28.26 184.47,28.26 182.56,26.35 167.96,26.35 167.32,25.72 v163.19,25.72 | IC23.42 92.71,46.99 99.06,46.99 100.33,45.72 100.33,40.64 102.87,38.1 v140.97,38.1 | v140.97,33.66 154.94,33.66 155.89,32.7 v163.19,32.7
N$215  (via drill 0.6)
  Top 0.406: OK9.6 RN3.7 IC18.7 v196.85,37.47
  Bottom 0.406: v196.85,37.47 179.7,37.47 179.07,38.1 177.48,38.1 176.85,37.47 165.73,37.47 165.1,36.83 157.48,36.83 154.94,39.37 148.59,39.37 147.32,40.64 102.87,40.64 101.6,41.91 101.6,46.99 100.33,48.26 IC23.44
N$216
  Top 0.406: IC18.6 RN3.6 194.31,29.21 196.21,27.31 197.48,27.31 198.12,26.04 OK9.7
  Bottom 0.406: JP1.2 177.8,31.75 193.04,31.75 RN3.6
N$217
  Top 0.406: IC18.5 RN3.5 191.77,29.21 190.5,27.94 189.23,27.94 187.96,26.67 OK6.10
N$218
  Top 0.406: IC18.4 RN3.4 189.23,29.21 186.69,26.67 184.15,26.67 OK6.12
N$219
  Top 0.406: IC18.3 RN3.3 185.42,29.21 184.15,29.21 181.61,26.67 179.07,26.67 OK6.14
N$220  (via drill 0.6)
  Top 0.406: IC18.2 RN3.2 | OK6.16 173.99,26.67 175.58,26.67 v176.85,27.94 | v162.56,24.13 v162.56,7.94
  Bottom 0.406: v176.85,27.94 181.61,27.94 RN3.2 | OK6.16 168.91,25.4 167.64,24.13 v162.56,24.13 | v162.56,7.94 162.24,7.62 149.86,7.62 IC15.32
N$221  (via drill 0.6)
  Top 0.406: v219.39,81.28 219.39,46.67 218.44,45.72 v218.44,29.21 | v154.94,20.32 154.94,7.62 IC15.35 | U$2.A 60.96,43.82 61.59,44.45 62.23,44.45 | v67.95,62.23 69.22,60.96 IC23.16 | v67.95,46.36 66.04,44.45 62.23,44.45 | 62.23,44.45 62.23,40.01 62.86,39.37 67.95,39.37 68.58,38.74 68.58,33.02 72.39,29.21 v73.66,29.21 | v97.16,28.58 v97.16,24.77
  Bottom 0.406: IC21.1 v219.39,81.28 | v218.44,29.21 184.15,29.21 181.93,26.99 163.51,26.99 162.88,26.35 153.67,26.35 | 153.67,26.35 IC15.11 154.94,22.86 v154.94,20.32 | v67.95,46.36 v67.95,62.23 | v73.66,29.21 96.52,29.21 v97.16,28.58 | v97.16,24.77 121.6,24.77 123.19,26.35 153.67,26.35
N$222  (via drill 0.6)
  Top 0.406: v164.15,21.59 v164.15,33.66
  Bottom 0.406: IC18.1 180.34,33.02 175.26,33.02 174.31,33.66 v164.15,33.66 | IC15.6 v164.15,21.59
N$223  (via drill 0.6)
  Top 0.406: v176.53,97.79 176.53,62.23 175.89,61.6 v175.89,38.42 | v160.02,38.1 160.02,25.4 IC15.7
  Bottom 0.406: IC17.1 v176.53,97.79 | v160.02,38.1 161.61,38.1 162.24,38.42 v175.89,38.42
N$224  (via drill 0.6)
  Top 0.406: v135.89,13.97 v135.89,5.72
  Bottom 0.406: RN5.3 SV1.1 120.65,12.7 123.19,12.7 124.46,13.97 v135.89,13.97 | v135.89,5.72 136.52,5.08 149.86,5.08 IC15.33
N$225  (via drill 0.6)
  Top 0.406: v130.81,7.62 130.81,13.65 131.13,13.97 131.13,20.64 v130.81,20.96 | v134.94,19.05 138.75,19.05 140.02,20.32 149.86,20.32 IC15.14
  Bottom 0.406: RN5.5 115.57,8.89 116.84,7.62 120.65,7.62 SV1.6 125.73,8.89 127,7.62 v130.81,7.62 | v130.81,20.96 131.44,20.96 133.35,19.05 v134.94,19.05
N$226  (via drill 0.6)
  Top 0.406: v116.84,5.08 116.84,7.62 118.11,8.89 SV1.5 | v123.83,24.45 123.83,20.64 124.78,19.69 124.78,10.8 v125.41,10.16
  Bottom 0.406: RN5.7 115.57,3.81 v116.84,5.08 | SV1.5 120.65,10.16 v125.41,10.16 | IC15.13 149.86,25.4 124.78,25.4 v123.83,24.45
N$227
  Top 0.406: OK6.3 177.8,16.51 179.07,15.24 185.42,15.24 R105.1
N$228  (via drill 0.6)
  Top 0.406: RN5.6 109.22,5.08 109.22,2.54 149.86,2.54 152.4,5.08 152.4,7.62 IC15.36
  Bottom 0.406: SV1.3 118.11,11.43 116.84,10.16 109.22,10.16 109.22,7.62 RN5.6
  other vias: 110.49,6.35
N$229  (via drill 0.6)
  Top 0.406: v139.7,13.97 v139.7,7.62
  Bottom 0.406: RN5.4 107.95,10.16 107.95,6.35 110.49,5.08 113.03,5.08 114.3,6.35 SV1.7 120.65,5.08 133.35,5.08 135.89,7.62 v139.7,7.62 | IC15.24 v139.7,13.97
N$230
  Bottom 0.406: OK6.5 182.88,16.51 183.83,15.56 190.18,15.56 R106.1
N$231
  Top 0.406: OK6.7 187.96,16.51 188.59,15.88 196.21,15.88 196.85,15.24 R107.1
N$232  (via drill 0.6)
  Top 0.406: OK6.8 191.77,16.51 196.85,16.51 OK9.2
  Top 0.61: OK6.6 185.42,16.51 180.34,16.51 OK6.4 | K3.16 D35.A 228.6,8.89 v228.6,3.81
  Top 1.016: OK6.2 175.26,10.16 176.53,8.89 X7.1
  Bottom 0.406: OK9.2 199.39,16.51 200.66,16.51 | OK9.3 200.66,16.51 | 200.66,16.51 210.82,16.51 | OK7.2 210.82,16.51 | 210.82,16.51 212.72,16.51 213.36,17.15 | 213.36,17.15 OK7.3 | R113.1 220.98,16.51 213.99,16.51 213.36,17.15
  Bottom 0.61: OK6.2 175.26,16.83 175.58,16.51 180.02,16.51 180.34,16.83 OK6.4 | OK6.6 185.42,17.15 186.05,16.51 189.86,16.51 190.5,17.15 OK6.8 | v228.6,3.81 228.6,1.27 | 252.73,120.65 248.28,120.65 247.65,121.28 OK4.4 | OK4.2 252.73,120.65 | OK5.4 261.62,120.65 | 261.62,120.65 266.7,120.65 | 266.7,120.65 OK5.2 | 252.73,120.65 261.62,120.65 | 266.7,120.65 270.51,120.65 271.78,119.38 280.67,119.38 281.94,118.11 281.94,60.96 289.56,53.34 295.91,53.34 297.18,52.07 302.26,52.07 303.53,50.8 307.34,50.8 309.88,48.26 309.88,40.64 311.15,39.37 321.31,39.37 326.39,34.29 334.01,34.29 334.8,33.5 X12.6
  Bottom 1.016: X6.9 196.54,1.28 | 196.54,1.28 195.26,1.27 178.43,1.27 X7.1 | 196.54,1.28 196.56,1.27 228.6,1.27 320.04,1.27 321.31,2.54 321.31,15.24 323.85,17.78 331.47,17.78 333.53,19.84 X12.9 X12.8 X12.7 X12.6
N$233
  Top 0.406: OK9.4 203.2,16.51 205.74,15.24 207.01,15.24 R108.1
N$234
  Bottom 0.406: R109.1 201.93,15.24 201.29,15.88 196.85,15.88 195.58,17.15 OK9.1
N$235
  Top 0.406: OK7.4 217.17,17.78 R110.1
N$236
  Top 0.406: OK7.1 210.82,15.24 212.09,15.24 R111.1
N$237
  Bottom 0.406: R107.2 199.39,12.7 200.66,11.43 202.88,11.43 206.06,8.26 X6.1
N$238  (via drill 0.6)
  Top 1.016: X7.2 181.61,2.54 182.88,1.27 198.12,1.27 199.39,2.54 199.39,3.56 X6.8 | 280.67,1.27 207.16,1.27 X6.6 | 280.67,1.27 280.67,5.08 281.94,6.35 282.02,6.35 X10.5 | v321.31,20.32 321.31,2.54 320.04,1.27 280.67,1.27
  Bottom 0.61: OK8.8 318.77,27.94
  Bottom 1.016: X6.8 X6.7 X6.6 | 327.66,27.94 327.66,20.55 X12.5 | 327.66,27.94 321.31,27.94 | 327.66,27.94 328.3,28.58 328.3,30.48 329.56,31.75 330.45,31.75 X12.1 | OK8.6 313.69,27.94 318.77,27.94 321.31,27.94 | 321.31,27.94 v321.31,20.32
N$239
  Bottom 0.406: R106.2 195.58,12.7 196.85,12.7 200.66,8.89 201.93,8.89 203.2,7.62 X6.2
N$240
  Bottom 0.406: R105.2 189.23,12.7 194.31,12.7 194.94,12.07 195.9,12.07 200.66,7.3 X6.3
N$241
  Bottom 0.406: R104.2 184.15,12.07 185.1,11.11 194.94,11.11 196.85,9.21 196.85,8.26 197.8,7.3 X6.4
N$242
  Bottom 0: X9.8 231.7,6.43 231.77,6.35
  Bottom 0.406: R109.2 204.47,12.7 207.01,10.16 230.5,10.16 231.77,8.89 231.77,6.35
N$243
  Bottom 0.406: R108.2 209.55,12.7 210.82,11.43 232.09,11.43 234.31,9.21 234.31,6.63 X9.7
N$244
  Bottom 0.406: R110.2 221.3,12.38 234,12.38 237.17,9.21 237.17,6.52 X9.6
N$245
  Top 1.016: K1.S2 255.91,17.15 268.61,17.15 271.78,13.97 282.57,13.97 288.29,8.26 X10.3
  Bottom 1.016: X9.5 X9.4 | X9.4 X9.12 | X9.4 242.67,7.72 250.19,15.24 254,15.24 K1.S2 | X10.3 289.56,8.89 291.47,10.8 316.23,10.8 318.13,8.89 X8.2
N$246  (via drill 0.6)
  Top 0.406: v240.03,11.43 255.27,11.43 259.72,15.88 267.97,15.88 274.96,8.89 283.79,8.89 X10.4
  Bottom 0.406: R111.2 215.9,15.24 222.25,15.24 R113.2 224.79,13.97 236.22,13.97 238.76,11.43 v240.03,11.43
N$247
  Bottom 0.406: X9.9 X9.10
N$248  (via drill 0.6)
  Top 1.016: D34.A 252.73,53.34 251.46,54.61 251.46,58.42 252.73,59.69 254,59.69 254,62.23 255.27,63.5 IC22.11
  Bottom 1.016: K1.1 254,46.99 D34.A
  other vias: 252.73,48.26
N$249
  Top 1.016: K1.P1 247.65,24.13 248.92,25.4 248.92,41.91 K1.2
  Bottom 1.016: D34.C 246.38,46.99 K1.2 246.38,40.64 K3.S1
N$250  (via drill 0.6)
  Top 1.016: K1.P2 256.54,25.4 256.54,35.56 259.08,38.1 283.21,38.1 v286.38,34.93 | X10.1 293.37,6.91 293.37,19.05 v292.1,19.05
  Bottom 1.016: v286.38,34.93 289.56,31.75 289.56,21.59 v292.1,19.05
N$251  (via drill 0.6)
  Top 0.406: R93.1 273.05,107.95 265.43,100.33 v265.43,97.79
  Top 1.016: C58.+ 255.59,56.52 255.27,56.2 257.49,56.2 SV2.1
  Bottom 0.406: IC22.10 257.81,60.96 259.08,62.23 259.08,73.66 260.35,74.93 265.43,74.93 266.7,76.2 266.7,92.71 265.43,93.98 v265.43,97.79 | R114.1 314.96,38.1 312.42,38.1 R115.1 304.8,43.18 K5.1
  Bottom 1.016: K5.1 304.8,48.26 D38.C 302.26,49.53 300.99,50.8 295.91,50.8 294.64,52.07 287.02,52.07 279.4,59.69 256.54,59.69 | K3.P1 241.3,24.13 243.84,21.59 | K1.S1 243.84,21.59 | 243.84,21.59 243.84,31.75 247.65,35.56 257.81,35.56 | K2.S1 265.43,19.05 265.43,30.48 260.35,35.56 257.81,35.56 | 257.81,35.56 SV2.1 257.81,57.15 256.54,59.69 | 256.54,59.69 IC22.10
N$252  (via drill 0.6)
  Top 0.406: X6.5 195.17,7.21 196.85,8.89 222.25,8.89 v229.87,16.51
  Bottom 0.406: v229.87,16.51 237.49,16.51 D35.C
  Bottom 0.813: D35.C K3.1
N$253
  Bottom 0.406: OK1.2 279.4,106.68 267.97,106.68 259.08,97.79 259.08,88.9 256.54,86.36 IC22.18
N$254
  Top 1.016: K2.P1 267.97,19.05 K2.S2
N$255
  Bottom 1.016: K2.P2 275.59,19.05 K4.S1
N$256  (via drill 0.6)
  Top 1.016: K2.2 264.8,46.36 277.5,46.36 K4.2 281.94,41.91 288.29,41.91 289.56,40.64 v289.56,39.37 | R112.2 298.45,26.67 300.99,24.13 300.99,16.51 308.61,12.7 v313.06,12.7 X8.1
  Bottom 0.61: D37.A K2.2
  Bottom 1.016: D36.A 279.4,45.72 K4.2 | v289.56,39.37 289.56,35.56 292.1,33.02 R112.2 | X11.2 270.51,6.99 272.42,8.89 287.02,8.89 290.83,12.7 v313.06,12.7 | X10.9 X10.8 X10.7 X10.6 297.03,3.66 298.45,5.08 298.45,7.62 299.72,8.89 309.88,8.89 313.06,5.08 X8.1
N$257
  Top 1.016: K4.S2 288.29,20.32 295.91,20.32 K5.S1
  Bottom 1.016: K5.S1 297.18,16.51 295.28,14.61 290.19,14.61 286.38,10.8 254.63,10.8 250.9,7.06 X9.1
N$258  (via drill 0.6)
  Top 1.016: v264.8,14.61 X11.1
  Bottom 0.406: D39.A 289.56,44.45 K4.1
  Bottom 1.016: D36.C K4.1 287.02,43.18 283.85,40.64 283.85,26.67 K4.P2 283.85,21.59 283.85,17.15 282.57,14.61 v264.8,14.61
N$259  (via drill 0.6)
  Top 1.016: X10.2 291.03,8.69 283.21,16.51 283.21,33.02 280.67,35.56 v270.51,35.56
  Bottom 0.61: D37.C 270.51,45.72 K2.1
  Bottom 1.016: K2.1 v270.51,35.56
N$260
  Bottom 1.016: K5.P1 294.64,21.59 294.64,18.42 293.37,17.15 290.19,17.15 285.75,12.7 251.46,12.7 248.16,9.4 X9.2
N$261  (via drill 0.6)
  Top 0.406: v276.86,58.42 273.05,58.42 271.78,59.69 271.78,62.23 266.7,67.31 266.7,73.66 261.62,78.74 IC22.17
  Bottom 0.406: v276.86,58.42 284.48,50.8 293.37,50.8 293.37,46.99 297.18,46.99
  Bottom 0.61: K5.2 297.18,46.99 D38.A
N$262
  Bottom 0.406: D39.K R112.1
N$263
  Bottom 0.406: R114.2 OK8.1
N$264
  Top 0.406: D42.K 260.35,74.93 259.08,76.2 IC22.16
N$265
  Bottom 0.406: D41.K 259.08,80.01 257.81,78.74 257.81,74.93 IC22.15
N$266
  Top 0.406: OK8.2 314.96,34.29 311.15,34.29 308.61,36.83 308.61,38.1 304.8,41.91 303.53,41.91 302.26,43.18 302.26,45.72 300.99,46.99 297.18,46.99 292.1,52.07 273.05,52.07 270.51,54.61 270.51,60.96 265.43,66.04 265.43,67.31 257.81,67.31 IC22.13
N$267
  Top 0.406: OK8.4 310.52,33.02 306.71,36.83 306.71,38.74 304.17,41.28 297.18,41.28 294.64,43.82 294.64,48.26 291.47,51.44 272.42,51.44 269.24,54.61 269.24,59.69 264.16,64.77 264.16,66.04 IC22.12
N$268  (via drill 0.6)
  Top 1.016: K6.3 281.94,102.87 281.94,88.9 | K7.3 281.94,88.9 | 281.94,88.9 281.94,71.12 K8.3 | K10.A1 279.4,62.46 279.4,57.79 v276.86,55.25
  Bottom 0.406: D44.C 279.4,74.93 K8.3 | D43.C 273.05,86.36 274.19,85.22 K9.A1 | R116.2 276.83,64.77 K10.A1
  Bottom 1.016: K7.3 K9.A1 | K8.3 K10.A1 | v276.86,55.25 276.86,26.67 K4.P1
N$269
  Bottom 0.406: D40.K 264.16,92.71 265.43,91.44 265.43,77.47 264.16,76.2 260.35,76.2 257.81,73.66 257.81,72.39 IC22.14
N$270
  Top 0.406: 270.51,88.9 D43.A
  Top 0.61: K7.4 270.51,88.9 265.43,88.9 260.35,83.82 D41.A
  Bottom 1.016: K9.A2 K7.4
N$271
  Bottom 0.406: K10.A2 275.59,72.46 D44.A | D42.A 273.05,69.85 K8.4
  Bottom 1.016: K10.A2 K8.4
N$272
  Bottom 0.813: 292.1,92.71 292.1,92.78 K9.22
  Bottom 2.184: K9.11 297.12,92.71 | K9.21 297.12,92.71 | 297.12,92.71 292.1,92.71 K7.2 | K9.22 292.08,104.14 K6.2 296.93,108.97 F2.1A F2.1B
N$273
  Bottom 0.406: K6.4 269.24,104.14 D40.A
N$274
  Bottom 0.813: 302.16,88.9 K7.1
  Bottom 2.184: K9.24 302.16,88.9 K9.14 | X13.6 323.85,81.28 320.04,83.82 R119.1 317.5,87.63 304.8,87.63 K7.1
N$275
  Bottom 2.184: 297.12,68.58 K8.2 | 297.12,68.58 K10.21 297.12,73.6 299.72,76.2 313.69,76.2 | 297.12,68.58 K10.11 | X13.7 313.69,76.2 | R118.1 313.69,76.2
N$276
  Bottom 1.676: 302.16,68.58 K8.1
